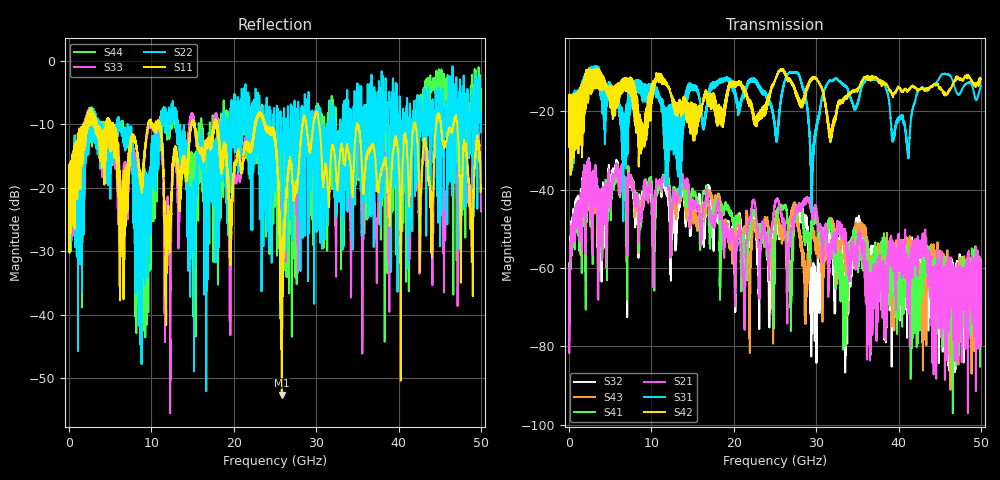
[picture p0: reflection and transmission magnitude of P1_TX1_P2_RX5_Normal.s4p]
!Keysight Technologies,N5225B,MY57041031,A.13.20.10
!Date: Friday, May 31, 2019 11:34:59
!Correction: S11(Full 4 Port(1,2,3,4))
!S12(Full 4 Port(1,2,3,4))
!S13(Full 4 Port(1,2,3,4))
!S14(Full 4 Port(1,2,3,4))
!S21(Full 4 Port(1,2,3,4))
!S22(Full 4 Port(1,2,3,4))
!S23(Full 4 Port(1,2,3,4))
!S24(Full 4 Port(1,2,3,4))
!S31(Full 4 Port(1,2,3,4))
!S32(Full 4 Port(1,2,3,4))
!S33(Full 4 Port(1,2,3,4))
!S34(Full 4 Port(1,2,3,4))
!S41(Full 4 Port(1,2,3,4))
!S42(Full 4 Port(1,2,3,4))
!S43(Full 4 Port(1,2,3,4))
!S44(Full 4 Port(1,2,3,4))
!S4P File: Measurements: <S11,S12,S13,S14>,
!<S21,S22,S23,S24>,
!<S31,S32,S33,S34>,
!<S41,S42,S43,S44>:
# Hz S  dB  R 50.0
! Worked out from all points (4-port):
!   5000 points, 10 MHz to 50 GHz, reference 50 ohm
!   strongest paths, dB at 10 MHz, 12.51 GHz, 25.01 GHz, 37.51 GHz, 50 GHz:
!     S42: -19.5, -17.0, -12.0, -12.0, -11.9
!     S31: -19.4, -29.2, -24.6, -11.8, -13.5
!     S21: -60.5, -45.8, -43.6, -67.3, -79.7
!     S41: -62.2, -43.8, -54.2, -60.3, -63.0
!     S43: -63.6, -44.7, -48.3, -55.6, -64.5
!     S32: -62.5, -48.8, -48.4, -65.0, -63.6
!   lowest |S11| = -52.7 dB at 25.83 GHz (marker M1), VSWR 1.00, Z = 50 + j0.232 ohm
!   |S11| at or under -10 dB: 17.97 GHz to 22.61 GHz (4.636 GHz wide, 22.8 % of centre); 30.38 GHz to 34.95 GHz (4.565 GHz wide, 14 % of centre); 35 GHz to 41.82 GHz (6.815 GHz wide, 17.7 % of centre)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
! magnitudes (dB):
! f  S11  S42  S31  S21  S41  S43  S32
! 10 MHz  -19.9  -19.5  -19.4  -60.5  -62.2  -63.6  -62.5
! 5.74 GHz  -11.3  -18.3  -15.6  -33.3  -34.7  -33.8  -32.4
! 23.26 GHz  -8.2  -21.9  -14.6  -54.1  -50.3  -51.6  -54.5
! 25.83 GHz  -52.7  -9.4  -16.0  -47.2  -44.7  -53.8  -50.5
! 28.56 GHz  -8.6  -16.5  -15.0  -43.8  -53.0  -63.8  -48.5
! 29.93 GHz  -8.4  -11.5  -25.5  -44.8  -46.9  -53.0  -68.9
! 50 GHz  -19.6  -11.9  -13.5  -79.7  -63.0  -64.5  -63.6
